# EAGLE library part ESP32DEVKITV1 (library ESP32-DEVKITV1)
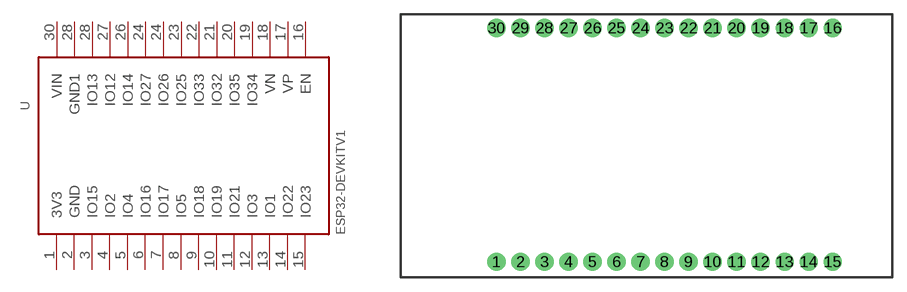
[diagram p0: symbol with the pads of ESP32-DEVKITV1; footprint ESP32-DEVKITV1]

Designator prefix -

## ESP32DEVKITV1  [ESP32-DEVKITV1]
1  3V3
2  GND
3  IO15
4  IO2
5  IO4
6  IO16
7  IO17
8  IO5
9  IO18
10  IO19
11  IO21
12  IO3
13  IO1
14  IO22
15  IO23
16  EN
17  VP
18  VN
19  IO34
20  IO35
21  IO32
22  IO33
23  IO25
24  IO26
24  IO27
26  IO14
27  IO12
28  IO13
28  GND1
30  VIN

## Footprint ESP32-DEVKITV1 (pad centres in mm)
drill 1 pad 1.93: 1 -22.87,-13.54; 2 -20.33,-13.54; 3 -17.79,-13.54; 4 -15.25,-13.54; 5 -12.71,-13.54; 6 -10.17,-13.54; 7 -7.63,-13.54; 8 -5.09,-13.54; 9 -2.55,-13.54; 10 -0.01,-13.54; 11 2.53,-13.54; 12 5.07,-13.54; 13 7.61,-13.54; 14 10.15,-13.54; 15 12.69,-13.54; 16 12.69,11.23; 17 10.15,11.23; 18 7.61,11.23; 19 5.07,11.23; 20 2.53,11.23; 21 -0.01,11.23; 22 -2.55,11.23; 23 -5.09,11.23; 24 -7.63,11.23; 25 -10.17,11.23; 26 -12.71,11.23; 27 -15.25,11.23; 28 -17.79,11.23; 29 -20.33,11.23; 30 -22.87,11.23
